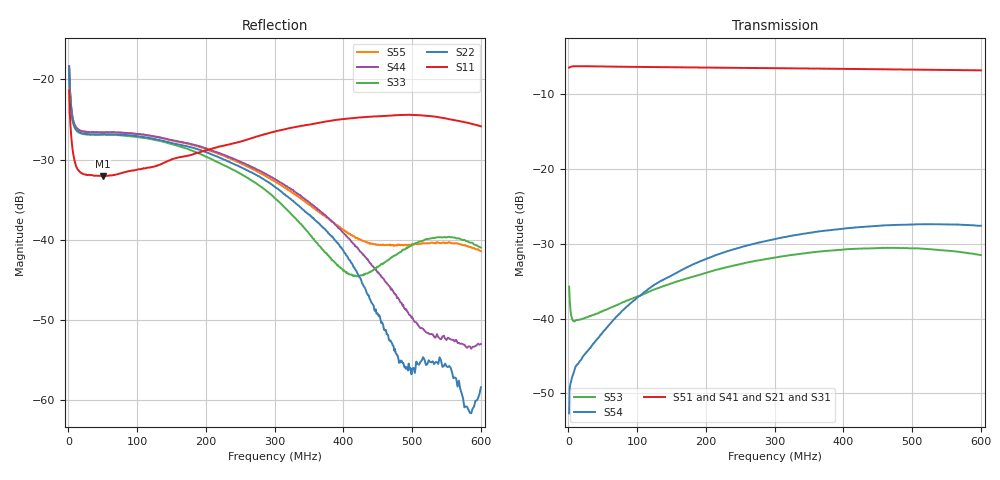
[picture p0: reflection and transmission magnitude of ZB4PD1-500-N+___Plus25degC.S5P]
!Mini-Circuits Laboratory
!S-Parameters
!MODEL:  ZB4PD1-500-N+
!Run/Lot/Date Code:H13510//
!DATA FOR:UNIT#1
!Fixture/SN/Due:N/A
!Connection:PORT-1= S11; PORT-2=S22;PORT-3=S33;PORT-4= S44;
!Created: 10-12-2010 at 10:44 AM
!S/N: Unit 1
#MHz S dB R 50
!Frequency  S11 dB  S11 DEG  S12 dB  S12 DEG  S13 dB  S13 DEG  S14 dB  S14 DEG  S15 dB  S15 DEG
!  S21 dB  S21 DEG  S22 dB  S22 DEG  S23 dB  S23 DEG  S24 dB  S24 DEG  S25 dB  S25 DEG
!  S31 dB  S31 DEG  S32 dB  S32 DEG  S33 dB  S33 DEG  S34 dB  S34 DEG  S35 dB  S35 DEG
!  S41 dB  S41 DEG  S42 dB  S42 DEG  S43 dB  S43 DEG  S44 dB  S44 DEG  S45 dB  S45 DEG
!  S51 dB  S51 DEG  S52 dB  S52 DEG  S53 dB  S53 DEG  S54 dB  S54 DEG  S55 dB  S55 DEG
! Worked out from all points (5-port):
!   550 points, 1 MHz to 600 MHz, reference 50 ohm
!   strongest paths, dB at 1 MHz, 138 MHz, 276 MHz, 413 MHz, 600 MHz:
!     S51: -6.5, -6.4, -6.6, -6.7, -6.9
!     S41: -6.5, -6.4, -6.6, -6.7, -6.9
!     S21: -6.5, -6.4, -6.6, -6.7, -6.9
!     S31: -6.5, -6.4, -6.6, -6.7, -6.9
!     S54: -52.7, -34.8, -29.9, -27.9, -27.6
!     S53: -35.7, -35.7, -32.2, -30.7, -31.5
!   lowest |S11| = -32.1 dB at 50 MHz (marker M1), VSWR 1.05, Z = 47.7 + j0.88 ohm
!   |S11| at or under -10 dB: start of sweep to end of sweep
